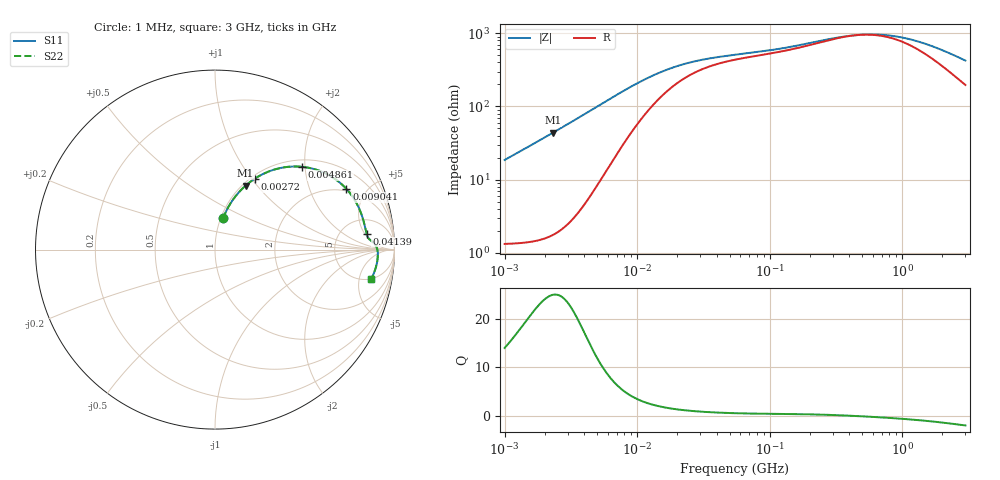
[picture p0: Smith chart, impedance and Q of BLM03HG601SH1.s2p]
! BLM03HG601SH1
# Hz S RI R 50
!Freq.(Hz) S11(Real) S11(Imag) S21(Real) S21(Imag) S12(Real) S12(Imag) S22(Real) S22(Imag)
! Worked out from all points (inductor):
!   401 points, 1 MHz to 3 GHz, reference 50 ohm
!   read as one part in series: L = 2.96 uH near 1.041 MHz
!   highest Q = 24.9 at 2.318 MHz (marker M1), where L = 3 uH
!   self-resonance near 469.8 MHz
!   S11 on the Smith chart (normalised r, x): 1 MHz: 1.03, +0.37; 2.72 MHz: 1.04, +1.04; 4.861 MHz: 1.15, +1.93; 9.041 MHz: 1.88, +3.64; 41.39 MHz: 9, +6; 3 GHz: 4.93, -7.50
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1000000  0.045 0.1745  0.955 -0.1745  0.955 -0.1745  0.045 0.1745
1584654  0.0911 0.2648  0.9089 -0.2648  0.9089 -0.2648  0.0911 0.2648
2317916  0.1706 0.3566  0.8294 -0.3566  0.8294 -0.3566  0.1706 0.3566
2720446  0.2209 0.3948  0.7791 -0.3948  0.7791 -0.3948  0.2209 0.3948
3823119  0.364 0.4544  0.636 -0.4544  0.636 -0.4544  0.364 0.4544
4861065  0.4846 0.4613  0.5154 -0.4613  0.5154 -0.4613  0.4846 0.4613
6831390  0.6423 0.4107  0.3577 -0.4107  0.3577 -0.4107  0.6423 0.4107
9040831  0.7326 0.3376  0.2674 -0.3376  0.2674 -0.3376  0.7326 0.3376
1.126754e7  0.7769 0.2787  0.2231 -0.2787  0.2231 -0.2787  0.7769 0.2787
1.461624e7  0.8077 0.2183  0.1923 -0.2183  0.1923 -0.2183  0.8077 0.2183
2.41077e7  0.8334 0.137  0.1666 -0.137  0.1666 -0.137  0.8334 0.137
4.138676e7  0.8445 0.0886  0.1555 -0.0886  0.1555 -0.0886  0.8445 0.0886
5.477226e7  0.8492 0.0739  0.1508 -0.0739  0.1508 -0.0739  0.8492 0.0739
1.148668e8  0.8667 0.0519  0.1333 -0.0519  0.1333 -0.0519  0.8667 0.0519
2.094008e8  0.8865 0.0353  0.1135 -0.0353  0.1135 -0.0353  0.8865 0.0353
3.252521e8  0.8984 0.0177  0.1016 -0.0177  0.1016 -0.0177  0.8984 0.0177
4.480278e8  0.9039 0.00241  0.0961 -0.00241  0.0961 -0.00241  0.9039 0.00241
6.049187e8  0.9066 -0.0135  0.0934 0.0135  0.0934 0.0135  0.9066 -0.0135
8.005644e8  0.9072 -0.0303  0.0928 0.0303  0.0928 0.0303  0.9072 -0.0303
1.059487e9  0.906 -0.0496  0.094 0.0496  0.094 0.0496  0.906 -0.0496
1.430499e9  0.9022 -0.0745  0.0978 0.0745  0.0978 0.0745  0.9022 -0.0745
3e9  0.8702 -0.1642  0.1298 0.1642  0.1298 0.1642  0.8702 -0.1642
